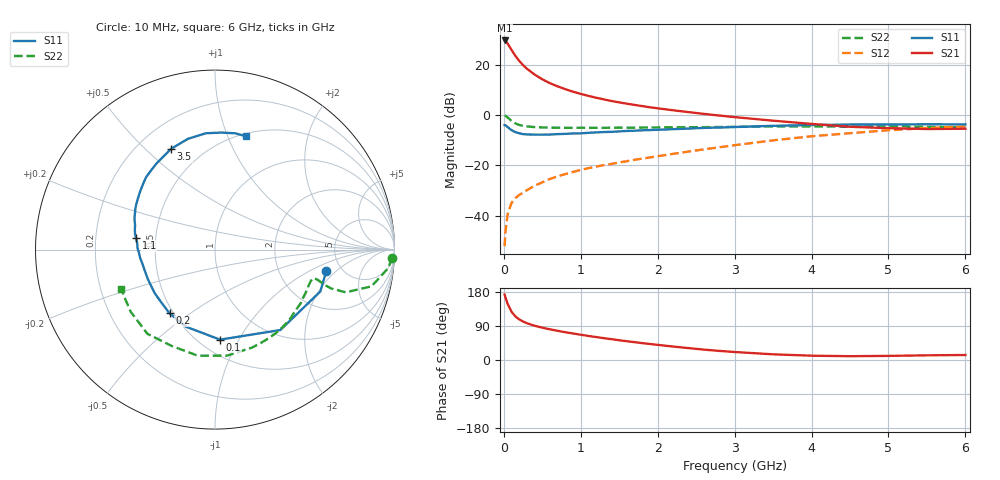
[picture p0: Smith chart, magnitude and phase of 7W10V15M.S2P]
! Infineon Technologies  Discrete & RF Semiconductors
! BFS17W
! Si NPN RF Bipolar Junction Transistor in SOT323
! VCE = 10 V  IC = 15 mA
! Common Emitter S-Parameters:  August  1999
# GHz  S  MA  R  50
!  f  S11  S21  S12  S22
! GHz  MAG  ANG  MAG  ANG  MAG  ANG  MAG  ANG
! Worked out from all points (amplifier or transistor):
!   36 points, 10 MHz to 6 GHz, reference 50 ohm
!   highest |S21| = 29.6 dB at 10 MHz (marker M1)
!   |S21| within 3 dB of that: start of sweep to 84.85 MHz
!   unconditionally stable (mu >= 1): 368.3 MHz to 2.051 GHz; 5.712 GHz to end of sweep
!   at 250 MHz: K = 0.88, MSG = 25.3 dB, |S12| = -30.8 dB
!   at 1.4 GHz: K = 1.15, MAG = 10.2 dB, |S12| = -19.4 dB
!   at 6 GHz: K = 1.02, MAG = -1.3 dB, |S12| = -4.5 dB
!   S11 on the Smith chart (normalised r, x): 10 MHz: 3.81, -1.49; 100 MHz: 0.62, -0.84; 200 MHz: 0.48, -0.42; 1.1 GHz: 0.39, +0.06; 3.5 GHz: 0.34, +0.60; 6 GHz: 0.53, +1.17
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0.01  0.6318 -10.7  30.35 172.8  0.0025 83.5  0.9867 -2.6
0.02  0.6315 -21.7  29.68 165.8  0.0047 79.1  0.9707 -6.1
0.05  0.5773 -50.9  26.29 147.7  0.0109 71.3  0.8959 -13.2
0.1  0.5025 -86.8  19.68 127.4  0.0181 61.0  0.7662 -18.1
0.15  0.4589 -110.5  15.02 114.9  0.0225 57.9  0.6827 -18.5
0.2  0.4364 -125.5  11.95 107.2  0.026 59.3  0.6388 -17.8
0.25  0.4187 -136.4  9.834 101.5  0.0287 59.4  0.6117 -16.9
0.3  0.4144 -144.2  8.329 97.1  0.0324 61.5  0.5963 -16.4
0.4  0.4089 -155.7  6.375 90.4  0.0396 63.3  0.5778 -16.1
0.5  0.4086 -163.3  5.144 85.3  0.0463 66.0  0.5699 -16.3
0.6  0.4117 -168.8  4.301 80.9  0.0541 67.1  0.5647 -17.1
0.7  0.4194 -173.5  3.717 77.0  0.061 68.5  0.5619 -18.2
0.9  0.4322 178.6  2.914 70.0  0.0744 69.5  0.5582 -21.2
1.1  0.445 171.6  2.407 63.4  0.0884 70.7  0.5593 -24.7
1.3  0.4612 165.6  2.052 57.6  0.1018 71.6  0.5592 -28.7
1.6  0.4849 157.5  1.682 49.5  0.1216 72.5  0.5622 -34.9
2.2  0.5255 143.0  1.247 35.5  0.1701 74.4  0.5731 -49.0
2.8  0.5672 128.9  0.981 24.0  0.2299 73.6  0.5801 -64.4
3.5  0.6126 113.5  0.775 15.0  0.3154 69.4  0.5946 -83.5
4.5  0.6502 94.5  0.587 10.0  0.4377 57.6  0.5886 -114.2
5.5  0.6578 80.2  0.529 12.3  0.5516 44.4  0.5836 -143.7
6  0.6547 74.6  0.536 13.2  0.597 37.7  0.5677 -157.1
